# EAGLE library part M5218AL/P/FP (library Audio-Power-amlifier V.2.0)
Dual power ampliefier
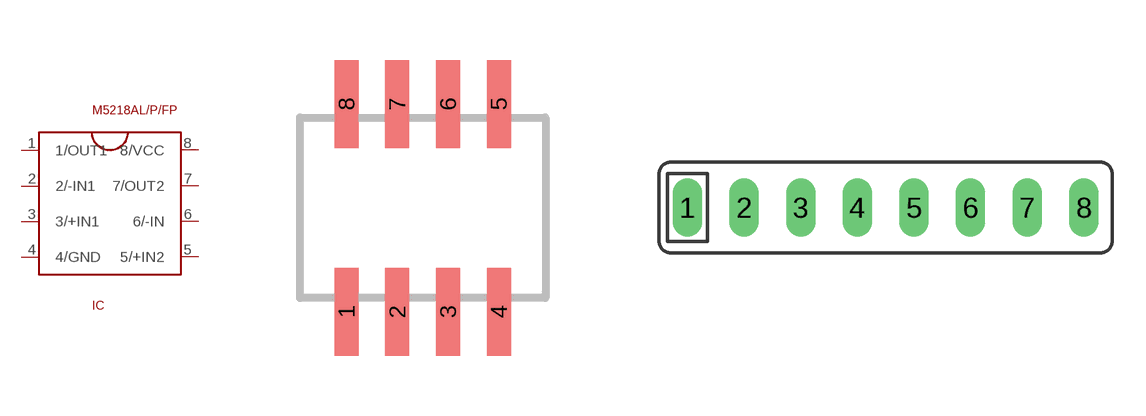
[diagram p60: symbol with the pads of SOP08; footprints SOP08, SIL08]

Designator prefix IC

## M5218AL/P/FP  [SOP08]
1  1/OUT1  out
2  2/-IN1  in
3  3/+IN1  in
4  4/GND  pwr
5  5/+IN2  in
6  6/-IN  in
7  7/OUT2  out
8  8/VCC  pwr

## M5218AL/P/FPSIL08  [SIL08]
Pads as for SOP08

## Footprint SOP08 (pad centres in mm)
smd 0.6 x 2.2: 1 -1.905,-2.6; 2 -0.635,-2.6; 3 0.635,-2.6; 4 1.905,-2.6; 5 1.905,2.6; 6 0.635,2.6; 7 -0.635,2.6; 8 -1.905,2.6

## Footprint SIL08 (pad centres in mm)
single in line 7 diodes with common anode
drill 0.813 long: 1 -8.89,0; 2 -6.35,0; 3 -3.81,0; 4 -1.27,0; 5 1.27,0; 6 3.81,0; 7 6.35,0; 8 8.89,0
